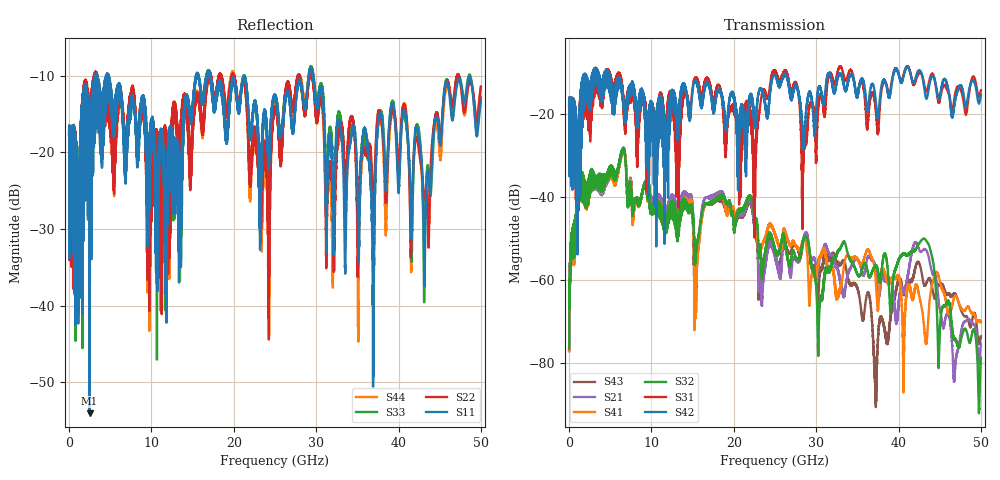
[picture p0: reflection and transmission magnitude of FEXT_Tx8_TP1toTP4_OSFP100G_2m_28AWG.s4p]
! Touchstone data
! Created: 27-Feb-2019 by IdEM 12 (12.1.0)
! COMMENTS
!  Created Wed Feb 27 12:03:36 2019
!  64 Port Network Data from SP1.SP block
!  freq  magS1_1  angS1_1  magS1_2  angS1_2  magS1_3  angS1_3  magS1_4  angS1_4
!  magS1_5  angS1_5  magS1_6  angS1_6  magS1_7  angS1_7  magS1_8  angS1_8
!  magS1_9  angS1_9  magS1_10  angS1_10  magS1_11  angS1_11  magS1_12  angS1_12
!  magS1_13  angS1_13  magS1_14  angS1_14  magS1_15  angS1_15  magS1_16  angS1_16
!  magS1_17  angS1_17  magS1_18  angS1_18  magS1_19  angS1_19  magS1_20  angS1_20
!  magS1_21  angS1_21  magS1_22  angS1_22  magS1_23  angS1_23  magS1_24  angS1_24
!  magS1_25  angS1_25  magS1_26  angS1_26  magS1_27  angS1_27  magS1_28  angS1_28
!  magS1_29  angS1_29  magS1_30  angS1_30  magS1_31  angS1_31  magS1_32  angS1_32
!  magS1_33  angS1_33  magS1_34  angS1_34  magS1_35  angS1_35  magS1_36  angS1_36
!  magS1_37  angS1_37  magS1_38  angS1_38  magS1_39  angS1_39  magS1_40  angS1_40
!  magS1_41  angS1_41  magS1_42  angS1_42  magS1_43  angS1_43  magS1_44  angS1_44
!  magS1_45  angS1_45  magS1_46  angS1_46  magS1_47  angS1_47  magS1_48  angS1_48
!  magS1_49  angS1_49  magS1_50  angS1_50  magS1_51  angS1_51  magS1_52  angS1_52
!  magS1_53  angS1_53  magS1_54  angS1_54  magS1_55  angS1_55  magS1_56  angS1_56
!  magS1_57  angS1_57  magS1_58  angS1_58  magS1_59  angS1_59  magS1_60  angS1_60
!  magS1_61  angS1_61  magS1_62  angS1_62  magS1_63  angS1_63  magS1_64  angS1_64
!  magS2_1  angS2_1  magS2_2  angS2_2  magS2_3  angS2_3  magS2_4  angS2_4
!  magS2_5  angS2_5  magS2_6  angS2_6  magS2_7  angS2_7  magS2_8  angS2_8
!  magS2_9  angS2_9  magS2_10  angS2_10  magS2_11  angS2_11  magS2_12  angS2_12
!  magS2_13  angS2_13  magS2_14  angS2_14  magS2_15  angS2_15  magS2_16  angS2_16
!  magS2_17  angS2_17  magS2_18  angS2_18  magS2_19  angS2_19  magS2_20  angS2_20
!  magS2_21  angS2_21  magS2_22  angS2_22  magS2_23  angS2_23  magS2_24  angS2_24
!  magS2_25  angS2_25  magS2_26  angS2_26  magS2_27  angS2_27  magS2_28  angS2_28
!  magS2_29  angS2_29  magS2_30  angS2_30  magS2_31  angS2_31  magS2_32  angS2_32
!  magS2_33  angS2_33  magS2_34  angS2_34  magS2_35  angS2_35  magS2_36  angS2_36
!  magS2_37  angS2_37  magS2_38  angS2_38  magS2_39  angS2_39  magS2_40  angS2_40
!  magS2_41  angS2_41  magS2_42  angS2_42  magS2_43  angS2_43  magS2_44  angS2_44
!  magS2_45  angS2_45  magS2_46  angS2_46  magS2_47  angS2_47  magS2_48  angS2_48
!  magS2_49  angS2_49  magS2_50  angS2_50  magS2_51  angS2_51  magS2_52  angS2_52
!  magS2_53  angS2_53  magS2_54  angS2_54  magS2_55  angS2_55  magS2_56  angS2_56
!  magS2_57  angS2_57  magS2_58  angS2_58  magS2_59  angS2_59  magS2_60  angS2_60
!  magS2_61  angS2_61  magS2_62  angS2_62  magS2_63  angS2_63  magS2_64  angS2_64
!  magS3_1  angS3_1  magS3_2  angS3_2  magS3_3  angS3_3  magS3_4  angS3_4
!  magS3_5  angS3_5  magS3_6  angS3_6  magS3_7  angS3_7  magS3_8  angS3_8
!  magS3_9  angS3_9  magS3_10  angS3_10  magS3_11  angS3_11  magS3_12  angS3_12
!  magS3_13  angS3_13  magS3_14  angS3_14  magS3_15  angS3_15  magS3_16  angS3_16
!  magS3_17  angS3_17  magS3_18  angS3_18  magS3_19  angS3_19  magS3_20  angS3_20
!  magS3_21  angS3_21  magS3_22  angS3_22  magS3_23  angS3_23  magS3_24  angS3_24
!  magS3_25  angS3_25  magS3_26  angS3_26  magS3_27  angS3_27  magS3_28  angS3_28
!  magS3_29  angS3_29  magS3_30  angS3_30  magS3_31  angS3_31  magS3_32  angS3_32
!  magS3_33  angS3_33  magS3_34  angS3_34  magS3_35  angS3_35  magS3_36  angS3_36
!  magS3_37  angS3_37  magS3_38  angS3_38  magS3_39  angS3_39  magS3_40  angS3_40
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# Hz S MA R 50
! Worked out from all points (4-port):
!   5000 points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, 10 MHz to 50 GHz, reference 50 ohm
!   strongest paths, dB at 10 MHz, 12.51 GHz, 25.01 GHz, 37.51 GHz, 50 GHz:
!     S42: -18.0, -15.9, -10.7, -20.7, -15.4
!     S31: -18.0, -16.4, -9.6, -24.1, -14.3
!     S32: -76.6, -44.9, -52.5, -58.2, -78.8
!     S41: -77.2, -44.7, -48.8, -67.1, -70.2
!     S21: -76.8, -42.8, -53.6, -62.8, -75.4
!     S43: -77.1, -43.3, -53.8, -74.7, -73.6
!   lowest |S11| = -54.1 dB at 2.49 GHz (marker M1), VSWR 1.00, Z = 49.8 + j0.0446 ohm
!   |S11| at or under -10 dB: 4.81 GHz to 15.41 GHz (10.6 GHz wide, 105 % of centre); 17.19 GHz to 29.09 GHz (11.9 GHz wide, 51.4 % of centre); 29.64 GHz to end of sweep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
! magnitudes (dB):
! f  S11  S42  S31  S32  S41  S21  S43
! 10 MHz  -17.7  -18.0  -18.0  -76.6  -77.2  -76.8  -77.1
! 2.49 GHz  -54.1  -17.4  -22.3  -40.1  -40.3  -40.0  -40.2
! 15.4 GHz  -10.2  -12.1  -11.1  -53.1  -61.6  -56.9  -63.5
! 21.94 GHz  -17.8  -16.6  -21.3  -40.0  -39.9  -40.9  -41.6
! 30.33 GHz  -12.9  -13.7  -17.2  -70.6  -54.7  -56.4  -61.4
! 43.16 GHz  -37.3  -14.3  -13.3  -50.1  -72.5  -52.6  -61.4
! 50 GHz  -13.3  -15.4  -14.3  -78.8  -70.2  -75.4  -73.6
